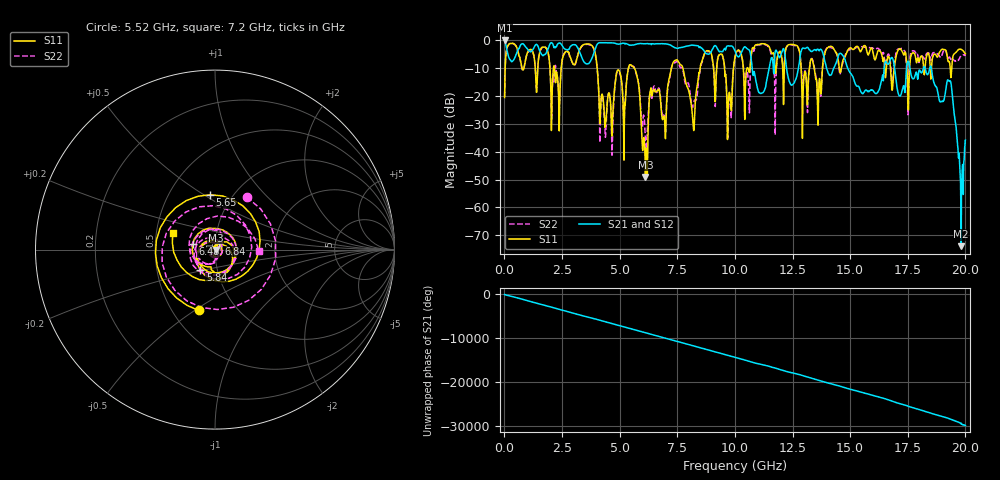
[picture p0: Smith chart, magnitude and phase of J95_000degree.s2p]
!Keysight Technologies,N5222A,MY51421036,A.10.65.16
!Date: Friday, March 31, 2023 14:16:02
!Correction: S11(Full 2 Port(1,2))
!S21(Full 2 Port(1,2))
!S12(Full 2 Port(1,2))
!S22(Full 2 Port(1,2))
!S2P File: Measurements: S11, S21, S12, S22:
# Hz S  dB  R 50
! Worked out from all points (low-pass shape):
!   2000 points, 10 MHz to 20 GHz, reference 50 ohm
!   highest |S21| = -0.18 dB at 10 MHz (marker M1); lowest = -73.9 dB at 19.82 GHz (marker M2)
!   |S21| within 3 dB of the highest: 1.897 GHz to 2.612 GHz (714.7 MHz wide, 31.7 % of centre); 3.941 GHz to 8.59 GHz (4.649 GHz wide, 74.2 % of centre)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
!   lowest |S11| = -49.1 dB at 6.12 GHz (marker M3), VSWR 1.01, Z = 50.3 - j0.144 ohm
!   |S11| at or under -10 dB: 4.026 GHz to 5.385 GHz (1.36 GHz wide, 28.9 % of centre); 5.63 GHz to 7.251 GHz (1.621 GHz wide, 25.2 % of centre); 7.74 GHz to 8.493 GHz (753 MHz wide, 9.28 % of centre)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
!   |S22| runs from -42.3 to -1.2 dB; largest |S21 - S12| = 0.014
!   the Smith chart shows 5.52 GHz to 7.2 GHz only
!   S11 on the Smith chart (normalised r, x): 5.52 GHz: 0.67, -0.52; 5.65 GHz: 0.79, +0.53; 5.84 GHz: 0.83, -0.19; 6.48 GHz: 0.78, +0.05; 6.84 GHz: 1.04, +0.07; 7.2 GHz: 0.61, +0.12
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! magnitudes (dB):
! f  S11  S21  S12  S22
! 10 MHz  -20.6  -0.2  -0.2  -20.4
! 3.35 GHz  -2.2  -6.1  -6.1  -2.4
! 4.37 GHz  -31.0  -1.0  -1.0  -33.8
! 5.52 GHz  -9.1  -1.8  -1.8  -9.3
! 5.65 GHz  -10.3  -1.7  -1.7  -10.1
! 5.84 GHz  -17.1  -1.3  -1.3  -16.5
! 6.12 GHz  -49.1  -1.3  -1.3  -37.5
! 6.48 GHz  -17.8  -1.4  -1.4  -16.7
! 6.68 GHz  -17.7  -1.4  -1.4  -17.3
! 6.84 GHz  -27.8  -1.3  -1.3  -26.9
! 7.2 GHz  -12.0  -1.8  -1.8  -12.2
! 8.19 GHz  -30.2  -1.9  -1.9  -23.1
! 8.68 GHz  -4.9  -4.1  -4.2  -5.0
! 9.4 GHz  -5.1  -4.2  -4.2  -5.3
! 9.76 GHz  -18.7  -2.2  -2.2  -19.6
! 10.01 GHz  -5.9  -4.0  -4.0  -6.4
! 11.13 GHz  -1.4  -19.2  -19.2  -1.7
! 13.34 GHz  -6.8  -4.1  -4.1  -6.6
! 16.67 GHz  -5.8  -8.6  -8.6  -5.1
! 19.3 GHz  -7.7  -14.8  -14.8  -6.1
! 19.82 GHz  -3.4  -73.9  -56.3  -5.7
! 20 GHz  -5.0  -35.9  -35.8  -5.7
